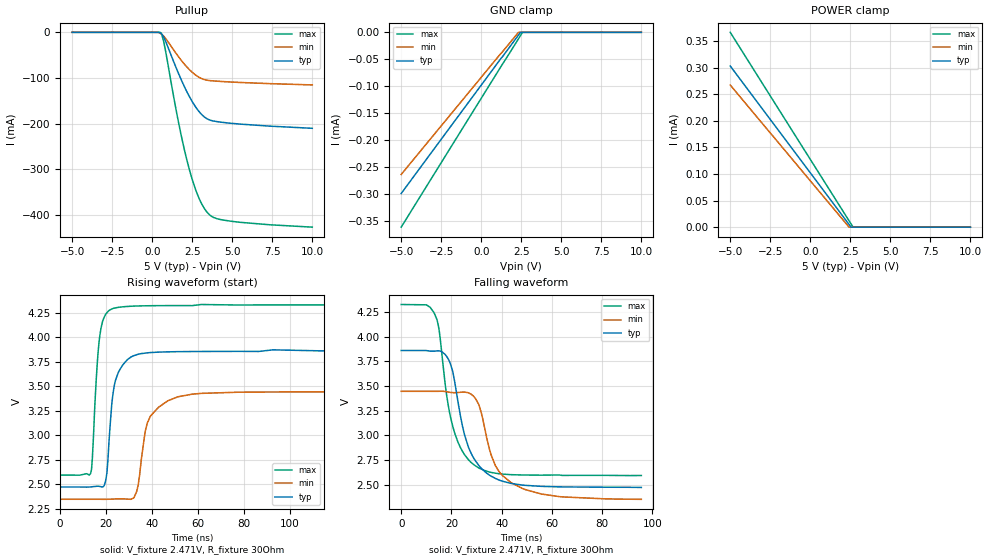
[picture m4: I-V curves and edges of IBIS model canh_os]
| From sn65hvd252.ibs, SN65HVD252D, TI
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|   canh_os Model
[Model]   canh_os
Model_type   Open_source
Polarity   Inverting
Vmeas = 3.17
Vref = 2.471
Cref = 100pF
Rref = 30
|   typ   min   max
|   (nom PVT)   (fast PVT)   (slow PVT)
C_comp   1.524e-11   1.524e-11   1.852e-11
| Where nom  PVT is Nominal Process, 5V, 27C
|   Fast PVT is Strong Process,  5.25V, -40C
|   Slow PVT is Weak Process,   4.75V, 125C
[Voltage Range]   5   4.75   5.25
|Ambient Temperature   25   85   -40
|Junction Temperature
[Temperature Range]   27   125   -40
[Pullup Reference]   5   4.75   5.25
[Pulldown Reference]   0   0   0
[Power Clamp Reference]   5   4.75   5.25
[GND Clamp Reference]   0   0   0
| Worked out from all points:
|   slope of the pullup table from 0 to 0.75 V, typ, clamps not added: 57.4 ohm
|   falling waveform, V_fixture 2.471V, R_fixture 30Ohm: 20-80 % time 8.37ns typ, 9.48ns min, 6.95ns max; typ from 3.86 V to 2.47 V
|   rising waveform, V_fixture 2.471V, R_fixture 30Ohm: 20-80 % time 3.65ns typ, 6.15ns min, 2.69ns max; typ from 2.47 V to 3.86 V
[GND Clamp]
|   Voltage   I(typ)   I(min)   I(max)
-5V       -298.7uA   -263.4uA   -361.1uA
2.325V    -5.125uA   -79.24nA   -12.03uA
2.45V     -91.52nA   0A         -6.043uA
2.576V    0A         0A         -46.73nA
10V       0A         0A         0A
[Pullup]
|   Voltage   I(typ)   I(min)   I(max)
-5V       0A         0A         0A
549.3mV   -2.331mA   -3.275mA   -1.381mA
723.8mV   -11.08mA   -8.727mA   -21.5mA
1.612V    -87.57mA   -51.93mA   -191.6mA
2.21V     -133.2mA   -77.53mA   -285.8mA
2.502V    -151.9mA   -87.58mA   -322.5mA
2.805V    -168.1mA   -95.86mA   -353.4mA
3.1V      -180.4mA   -101.5mA   -376.5mA
3.39V     -188.7mA   -104.7mA   -392.6mA
3.816V    -194.3mA   -106.4mA   -405.4mA
4.902V    -199.2mA   -108.8mA   -413.8mA
10V       -210.3mA   -115.2mA   -426.9mA
[POWER Clamp]
|   Voltage   I(typ)   I(min)   I(max)
-5V       303.1uA    267.3uA    366.4uA
2.42V     5.143uA    136.7nA    12.1uA
2.545V    109nA      0A         6.116uA
2.67V     0A         0A         144nA
10V       0A         0A         0A
[Ramp]
R_load = 30
|   typ   min   max
dV/dt_r   0.834098/3.67053e-09   0.660656/5.93359e-09   1.04088/2.67131e-09
dV/dt_f   0.833903/8.34283e-09   0.660374/9.44533e-09   1.04077/6.92637e-09
[Falling Waveform]
V_fixture = 2.471V
V_fixture_min = 2.346V
V_fixture_max = 2.593V
R_fixture = 30Ohm
|   Time   V(typ)   V(min)   V(max)
0s        3.861V     3.447V     4.328V
13.07ns   3.854V     3.447V     4.244V
14.98ns   3.857V     3.447V     4.087V
18.12ns   3.8V       3.443V     3.401V
20.6ns    3.636V     3.433V     3.084V
25.25ns   3.001V     3.439V     2.802V
29.6ns    2.74V      3.372V     2.69V
37.55ns   2.562V     2.69V      2.616V
43.75ns   2.512V     2.52V      2.601V
95.57ns   2.471V     2.351V     2.593V
[Rising Waveform]
V_fixture = 2.471V
V_fixture_min = 2.346V
V_fixture_max = 2.593V
R_fixture = 30Ohm
|   Time   V(typ)   V(min)   V(max)
0s        2.471V     2.346V     2.593V
13.25ns   2.472V     2.346V     2.609V
17.25ns   2.477V     2.346V     4.013V
20.32ns   2.613V     2.346V     4.247V
23.65ns   3.518V     2.349V     4.296V
33.25ns   3.82V      2.423V     4.317V
36.85ns   3.836V     3.016V     4.319V
39.23ns   3.842V     3.193V     4.32V
57.45ns   3.853V     3.418V     4.321V
349.9ns   3.861V     3.447V     4.328V
